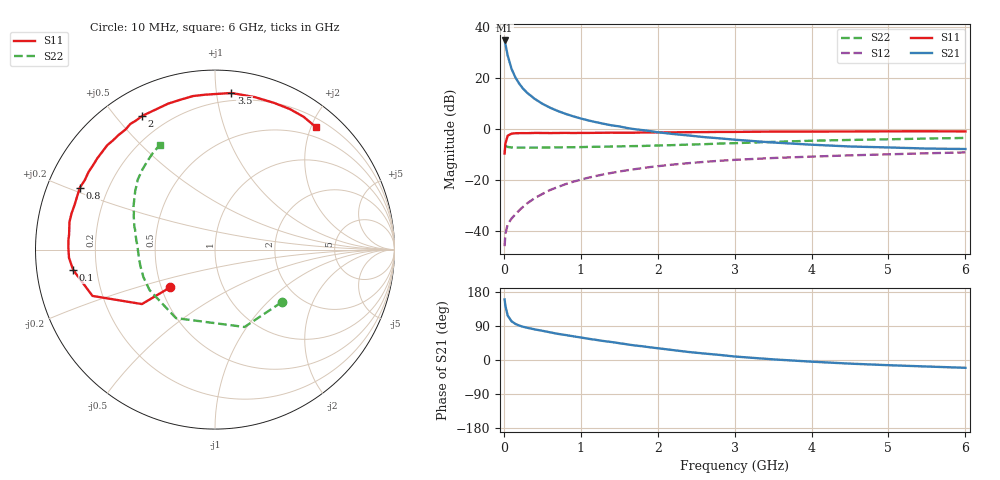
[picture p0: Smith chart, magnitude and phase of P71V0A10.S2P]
! SIEMENS Small Signal Semiconductors
! BFP196
! Si NPN RF Bipolar Junction Transistor in SOT143
! VCE = 1 V  IC = 100 mA
! Common Emitter S-Parameters:  May  1996
# GHz  S  MA  R  50
!  f  S11  S21  S12  S22
! GHz  MAG  ANG  MAG  ANG  MAG  ANG  MAG  ANG
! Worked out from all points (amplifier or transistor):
!   36 points, 10 MHz to 6 GHz, reference 50 ohm
!   highest |S21| = 34.6 dB at 10 MHz (marker M1)
!   |S21| within 3 dB of that: start of sweep to 30.72 MHz
!   unconditionally stable (mu >= 1): start of sweep to 15.17 MHz; 173.6 MHz to end of sweep
!   at 250 MHz: K = 1.11, MAG = 21.1 dB, |S12| = -30.6 dB
!   at 1.4 GHz: K = 1.18, MAG = 6.7 dB, |S12| = -17.3 dB
!   at 6 GHz: K = 1.08, MAG = -1.1 dB, |S12| = -9.3 dB
!   S11 on the Smith chart (normalised r, x): 10 MHz: 0.56, -0.26; 100 MHz: 0.11, -0.07; 800 MHz: 0.10, +0.22; 2 GHz: 0.11, +0.59; 3.5 GHz: 0.15, +1.10; 6 GHz: 0.33, +2.07
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0.01  0.3266 -139.9  53.47 159.7  0.005 62.9  0.4732 -38.3
0.02  0.5078 -143.3  45.5 143.1  0.0087 56.3  0.4615 -69.1
0.05  0.7298 -159.3  27.2 117.3  0.0133 45.4  0.4394 -119.7
0.1  0.7981 -171.8  14.85 102.1  0.0174 48.1  0.4288 -148.2
0.15  0.8148 -176.8  10.12 95.3  0.021 53.5  0.4273 -159.1
0.2  0.8171 179.1  7.631 90.8  0.0252 58.2  0.4254 -164.9
0.25  0.8183 176.3  6.08 87.7  0.0295 60.4  0.4255 -168.7
0.3  0.8173 174.0  5.092 85.2  0.0342 63.0  0.4255 -171.1
0.4  0.8252 169.3  3.849 80.9  0.0435 65.5  0.4263 -174.6
0.5  0.8245 165.9  3.086 77.1  0.0526 66.3  0.4277 -177.1
0.6  0.8211 162.2  2.58 73.1  0.0628 66.2  0.4287 -178.9
0.7  0.8234 158.8  2.225 69.1  0.0719 65.4  0.4303 179.4
0.8  0.8283 155.4  1.959 66.0  0.0818 64.4  0.4328 178.1
1.1  0.8262 145.4  1.448 56.0  0.1097 60.9  0.4395 174.2
1.6  0.8346 130.2  1.033 41.4  0.153 52.9  0.4536 168.4
2  0.8481 118.6  0.852 31.1  0.1841 46.1  0.4691 163.4
2.2  0.8473 113.2  0.787 26.1  0.1984 42.8  0.4768 161.0
3  0.8648 93.6  0.609 9.2  0.2454 29.8  0.5209 150.2
3.5  0.8774 84.0  0.536 1.7  0.2665 22.4  0.5511 143.8
4.5  0.8811 68.1  0.448 -9.6  0.3004 9.9  0.6021 132.2
5.5  0.8896 56.3  0.408 -17.2  0.3299 -1.0  0.6411 122.5
6  0.8842 50.7  0.4 -20.6  0.3431 -6.8  0.6596 117.6
